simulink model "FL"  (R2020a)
settings: Solver=VariableStepAuto  StartTime=0.0  StopTime=10.0  RelTol=1e-3
PreLoadFcn:
  | initParams
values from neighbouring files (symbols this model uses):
  b = 1    [initParams.m]
  g = 9.81    [initParams.m]
  K1 = 50    [initParams.m]
  K2 = 50    [initParams.m]
  m = 0.5    [initParams.m]
  R = 0.7    [initParams.m]
  x0 = [0.2;0.1]    [initParams.m]

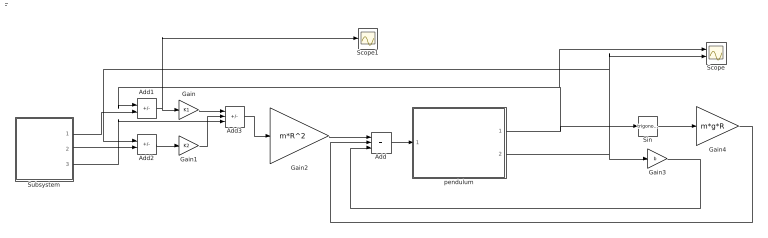
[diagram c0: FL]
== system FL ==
  Add : Sum  Inputs=+++
  Add1 : Sum  Inputs=+-
  Add2 : Sum  Inputs=+-
  Add3 : Sum  Inputs=--+
  Gain : Gain  Gain=K1
  Gain1 : Gain  Gain=K2
  Gain2 : Gain  Gain=m*R^2
  Gain3 : Gain  Gain=b
  Gain4 : Gain  Gain=m*g*R
  Scope : Scope  NumInputPorts=2
  Scope1 : Scope
  Sin : Trigonometry
  Subsystem : Subsystem
  pendulum : Subsystem
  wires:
  pendulum/1(theta) -> Scope/1, Add1/1, Sin/1
  Sin/1 -> Gain4/1
  pendulum/2(thetaDot) -> Scope/2, Add2/1, Gain3/1
  Gain2/1 -> Add/1
  Gain3/1 -> Add/3
  Gain4/1 -> Add/2
  Add/1 -> pendulum/1(tau)
  Subsystem/1(theta_d) -> Add1/2
  Add1/1 -> Scope1/1, Gain/1
  Add2/1 -> Gain1/1
  Subsystem/2(thetaDot_d) -> Add2/2
  Gain/1 -> Add3/1
  Add3/1 -> Gain2/1
  Gain1/1 -> Add3/2
  Subsystem/3(thetaDDot_d) -> Add3/3

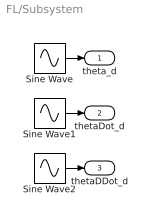
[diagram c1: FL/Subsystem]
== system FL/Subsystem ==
  Sine Wave : Sin  SampleTime=0
  Sine Wave1 : Sin  Phase=pi/2  SampleTime=0
  Sine Wave2 : Sin  Amplitude=-1  SampleTime=0
  theta_d : Outport
  thetaDot_d : Outport  Port=2
  thetaDDot_d : Outport  Port=3
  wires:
  Sine Wave/1 -> theta_d/1
  Sine Wave2/1 -> thetaDDot_d/1
  Sine Wave1/1 -> thetaDot_d/1

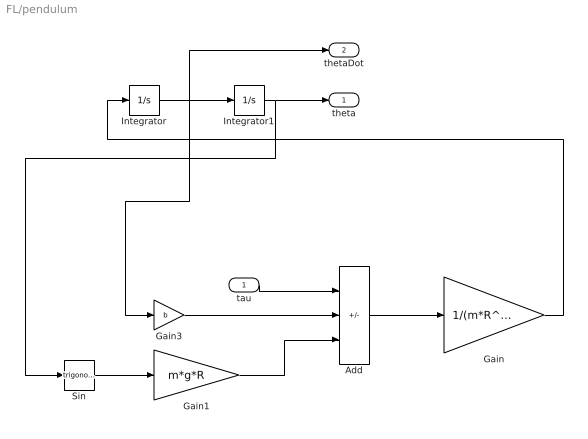
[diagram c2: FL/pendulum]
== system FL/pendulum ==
  tau : Inport
  Add : Sum  Inputs=+--
  Gain : Gain  Gain=1/(m*R^2)
  Gain1 : Gain  Gain=m*g*R
  Gain3 : Gain  Gain=b
  Integrator : Integrator  InitialCondition=x0(1)
  Integrator1 : Integrator  InitialCondition=x0(2)
  Sin : Trigonometry
  theta : Outport
  thetaDot : Outport  Port=2
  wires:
  Integrator/1 -> thetaDot/1, Gain3/1, Integrator1/1
  Sin/1 -> Gain1/1
  Integrator1/1 -> theta/1, Sin/1
  tau/1 -> Add/1
  Gain3/1 -> Add/2
  Add/1 -> Gain/1
  Gain1/1 -> Add/3
  Gain/1 -> Integrator/1
